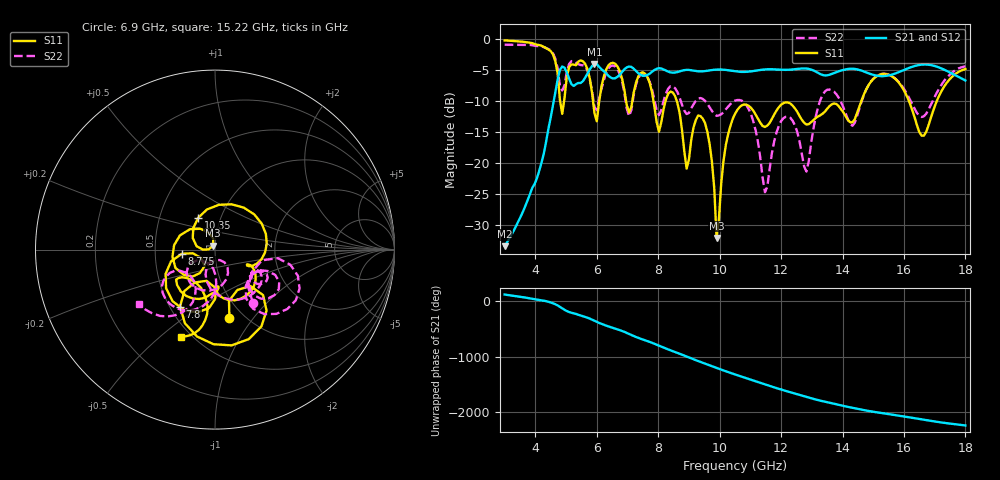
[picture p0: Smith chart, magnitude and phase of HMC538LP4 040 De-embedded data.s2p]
! Chelmsford, MA 01824
! http://www.hittite.com
! Tel: 978-250-3343
! Fax: 978-250-3373
! Device  :  HMC538LP4
! Description:  600 Analog Phase Shifter
! Frequency  :  6.0 GHz - 15.0 GHz
! Package  :  LP4  - 4x4 mm Quad Flatpack No-Lead (QFN) Plastic Package: 24 pin
! Ports  :  2 RF, 1 DC
!  Pin  3  = Rfin  = Port 1
!  Pin  16  = Rfout = Port 2
!  pin  21  = vCTL
! Voltages:  VCTL  = 0 to 5.0 Volts
! Currents :  Vb(V)  Vd(V)  Ib(mA)  Id(mA)
!  0.00  4.00  0.000000	0.482006
! Data:  The device was measured on evaluation board 111296-1.
!  Data was collected using a calibrated network analyzer.
!  The evaluation circuit board was modeled and simulated.This was use
!  to removed the evaluation board circuit from the measured data.
!  The reference plane is the center of the package pin.
! Misc:  Lot #
!Date Measured:  03 - 11 -2009
! Date:  03 - 17 -2009
! Note:
!  Hittite Microwave supplies this data as a sample of measured data at the
!  package pin for this package product.  Your particular data for this product
!  may vary.
!  Data was taken at 25 degrees C.
!  Hittite Microwave reserves the right to change this data at anytime.
# MHz S MA R 50
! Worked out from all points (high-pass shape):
!   201 points, 3 GHz to 18 GHz, reference 50 ohm
!   highest |S21| = -3.97 dB at 5.925 GHz (marker M1); lowest = -33.4 dB at 3 GHz (marker M2)
!   |S21| within 3 dB of the highest: 4.71 GHz to 5.152 GHz (442.3 MHz wide, 8.97 % of centre); 5.497 GHz to end of sweep
!   lowest |S11| = -32.0 dB at 9.9 GHz (marker M3), VSWR 1.05, Z = 48.9 + j2.24 ohm
!   |S11| at or under -10 dB: 7.847 GHz to 8.237 GHz (389.2 MHz wide, 4.84 % of centre); 8.606 GHz to 14.61 GHz (6.006 GHz wide, 51.7 % of centre); 16.16 GHz to 17.07 GHz (903.1 MHz wide, 5.44 % of centre)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
!   |S22| runs from -24.7 to -0.9 dB; largest |S21 - S12| = 0.0025
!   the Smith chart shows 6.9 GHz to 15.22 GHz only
!   S11 on the Smith chart (normalised r, x): 6.9 GHz: 0.86, -0.77; 7.8 GHz: 0.56, -0.42; 8.775 GHz: 0.69, -0.03; 10.35 GHz: 0.78, +0.29; 15.22 GHz: 0.44, -0.59
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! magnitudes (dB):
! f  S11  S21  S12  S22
! 3 GHz  -0.2  -33.4  -33.4  -0.9
! 4.8 GHz  -9.7  -4.9  -4.9  -7.5
! 5.55 GHz  -3.5  -6.8  -6.8  -4.2
! 5.925 GHz  -11.9  -4.0  -4.0  -10.9
! 6.9 GHz  -8.2  -4.8  -4.8  -8.7
! 7.8 GHz  -8.6  -5.2  -5.2  -8.1
! 8.025 GHz  -14.9  -4.7  -4.7  -12.2
! 8.4 GHz  -8.4  -5.3  -5.3  -7.6
! 8.775 GHz  -14.6  -5.1  -5.1  -10.6
! 8.925 GHz  -20.9  -4.9  -4.9  -12.1
! 9.525 GHz  -13.5  -5.1  -5.1  -9.9
! 9.9 GHz  -32.0  -4.9  -4.9  -12.4
! 10.35 GHz  -14.0  -5.1  -5.1  -10.5
! 10.5 GHz  -12.0  -5.2  -5.2  -9.9
! 11.47 GHz  -14.1  -4.9  -4.9  -24.7
! 12 GHz  -10.6  -4.9  -4.9  -13.2
! 12.82 GHz  -13.7  -4.7  -4.7  -21.3
! 13.05 GHz  -13.0  -5.0  -5.0  -14.5
! 15.22 GHz  -5.7  -5.9  -6.0  -5.6
! 15.53 GHz  -5.8  -5.8  -5.8  -5.7
! 16.65 GHz  -15.5  -4.1  -4.1  -12.4
! 18 GHz  -4.8  -6.6  -6.7  -4.4
